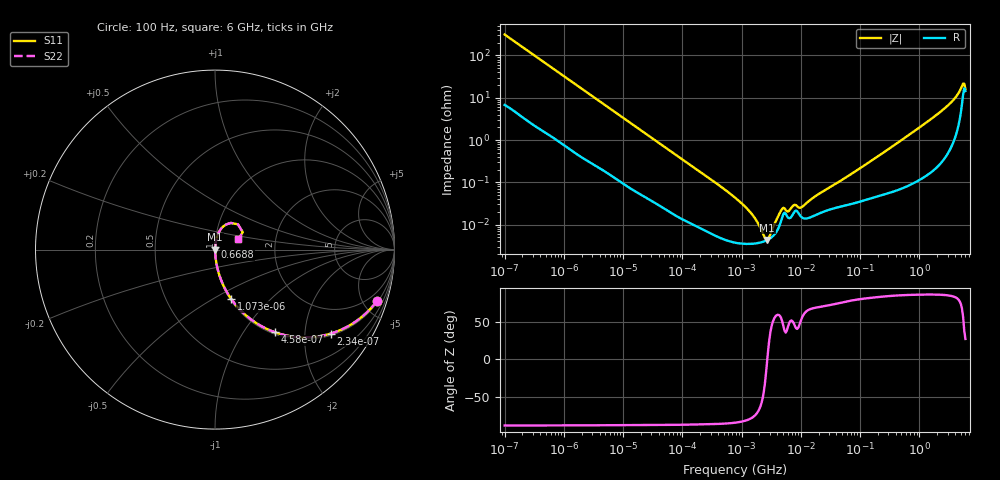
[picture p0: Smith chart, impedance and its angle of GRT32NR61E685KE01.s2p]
!Murata Part Number: GRT32NR61E685KE01
!These Parameters are Measured in Series Mode Connection
!Data Generated on Jun 19, 2026
!  o--ll--o
!Port1  Port2
!  o------o
!Operation Temp=25[degC], DC Bias Voltage=0[V]
!Freq. Start=100[Hz] Stop=6[GHz] 401[Steps]
# Hz S RI R 50
!Freq.(Hz) S11(Real) S11(Imag) S21(Real) S21(Imag) S12(Real) S12(Imag) S22(Real) S22(Imag)
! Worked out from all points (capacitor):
!   401 points, 100 Hz to 6 GHz, reference 50 ohm
!   read as one part in series: C = 5.05 uF near 109 Hz
!   lowest |Z| = 4.32 mohm at 2.714 MHz (marker M1)
!   series resonance near 2.717 MHz, so ESL is about 680 pH
!   S11 on the Smith chart (normalised r, x): 100 Hz: 1.14, -6.27; 234 Hz: 1.06, -2.71; 458 Hz: 1.03, -1.40; 1.073 kHz: 1.01, -0.61; 668.8 MHz: 1.00, +0.03; 6 GHz: 1.29, +0.15
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100  0.9026 -0.2859  0.0974 0.2859  0.0974 0.2859  0.9026 -0.2859
234  0.6452 -0.4677  0.3548 0.4677  0.3548 0.4677  0.6452 -0.4677
458  0.3322 -0.4599  0.6678 0.4599  0.6678 0.4599  0.3322 -0.4599
1073  0.0893 -0.2737  0.9107 0.2737  0.9107 0.2737  0.0893 -0.2737
2008  0.0295 -0.1577  0.9705 0.1577  0.9705 0.1577  0.0295 -0.1577
6433  0.00408 -0.0516  0.9959 0.0516  0.9959 0.0516  0.00408 -0.0516
40335  0.000358 -0.00855  0.9996 0.00855  0.9996 0.00855  0.000358 -0.00855
774597  3.76e-05 -0.000434  1 0.000434  1 0.000434  3.76e-05 -0.000434
1267578  3.5e-05 -0.000228  1 0.000228  1 0.000228  3.5e-05 -0.000228
1983483  3.72e-05 -8.83e-05  1 8.83e-05  1 8.83e-05  3.72e-05 -8.83e-05
2713602  4.32e-05 -3e-07  1 3e-07  1 3e-07  4.32e-05 -3e-07
3549919  5.73e-05 8.1e-05  0.9999 -8.1e-05  0.9999 -8.1e-05  5.73e-05 8.1e-05
4856642  0.00015 0.000184  0.9999 -0.000184  0.9999 -0.000184  0.00015 0.000184
6075234  0.000147 0.000141  0.9999 -0.000141  0.9999 -0.000141  0.000147 0.000141
7947587  0.000209 0.000207  0.9998 -0.000207  0.9998 -0.000207  0.000209 0.000207
1.039699e7  0.000148 0.000213  0.9999 -0.000213  0.9999 -0.000213  0.000148 0.000213
1.555665e7  0.000155 0.000386  0.9998 -0.000386  0.9998 -0.000386  0.000155 0.000386
3.124326e8  0.000602 0.00627  0.9994 -0.00627  0.9994 -0.00627  0.000602 0.00627
6.688484e8  0.00102 0.0132  0.999 -0.0132  0.999 -0.0132  0.00102 0.0132
3.8344e9  0.0174 0.0885  0.9826 -0.0885  0.9826 -0.0885  0.0174 0.0885
5.245841e9  0.0889 0.1486  0.9111 -0.1486  0.9111 -0.1486  0.0889 0.1486
6e9  0.1298 0.0566  0.8702 -0.0566  0.8702 -0.0566  0.1298 0.0566
